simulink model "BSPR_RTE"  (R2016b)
settings: Solver=FixedStepDiscrete  StartTime=0.0  StopTime=100.0  FixedStep=0.01  RelTol=1e-3  EnableMultiTasking=on
undefined symbols (not defined in the file): RTE_bDchrgDiagStdSel_C, RTE_tiBase_C, RTE_tiDebs_C, RTE_uDCWkUpLow_C, RTE_uDCWkUpUp_C
libraries: simulink x2

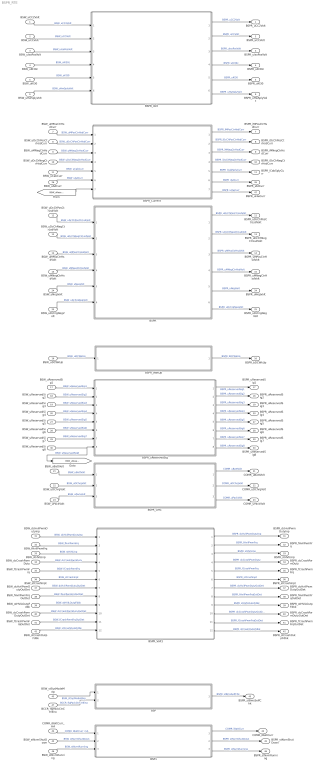
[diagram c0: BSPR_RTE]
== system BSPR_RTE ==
  BSW_uCC2Volt : Inport
  BSW_uCCVolt : Inport  Port=2
  BSW_uIsoPosVolt : Inport  Port=3
  BSW_uKl30c : Inport  Port=4
  BSW_uKl30 : Inport  Port=5
  BSW_uHwSplyVolt : Inport  Port=6
  BSW_uMPosCtrHsdCurr : Inport  Port=7
  BSW_uDcChPosCtrHsdCurr : Inport  Port=8
  BSW_uMNegCtrHsdCurr : Inport  Port=9
  BSW_uDcChNegCtrHsdCurr : Inport  Port=10
  BSW_uCabCurr : Inport  Port=11
  BSW_uDcChPosCtrLsdVolt : Inport  Port=12
  BSW_uDcChNegCtrLsdVolt : Inport  Port=13
  BSW_uMPosCtrHsdVolt : Inport  Port=14
  BSW_uMNegCtrHsdVolt : Inport  Port=15
  BSW_uDCWkUp : Inport  Port=16
  BSW_uReservedSig1 : Inport  Port=17
  BSW_uReservedSig2 : Inport  Port=18
  BSW_uReservedSig3 : Inport  Port=19
  BSW_uReservedSig4 : Inport  Port=20
  BSW_uBattVolt : Inport  Port=21
  BSW_uDChrgVolt : Inport  Port=22
  BSW_uPackVolt : Inport  Port=23
  BSW_uNegVolt : Inport  Port=24
  BSW_uDchrgNegVolt : Inport  Port=25
  BSW_uAdCurr : Inport  Port=26
  BSW_uReservedSig5 : Inport  Port=27
  BSW_uReservedSig6 : Inport  Port=28
  BSW_uReservedSig7 : Inport  Port=29
  BSW_uReservedSig8 : Inport  Port=30
  BSW_dcHvilPwmDutyInp : Inport  Port=31
  BSW_fHvilPwmFrq : Inport  Port=32
  BSW_stHVILInp : Inport  Port=33
  BSW_dcCrashPwmDuty : Inport  Port=34
  BSW_fCrashPwmFrq : Inport  Port=35
  BSW_stCrashInpt : Inport  Port=36
  BSW_dcHvilPwmDutyOutDet : Inport  Port=37
  BSW_fHvilPwmFrqOutDet : Inport  Port=38
  BSW_stHVILOutpFdbk : Inport  Port=39
  BSW_dcCrashPwmDutyOutDet : Inport  Port=40
  BSW_fCrashPwmFrqOutDet : Inport  Port=41
  BSW_stCrashOutpFdbk : Inport  Port=42
  BSW_stSysModeMag : Inport  Port=43
  " COMR_iBattCurr_mA" : Inport  Port=44
  " BSW_stNvmShutDown" : Inport  Port=45
  " BSW_stNvmRunning" : Inport  Port=46
  BCCR_flgPackCtrCtrlEna : Inport  Port=47
  BSP : Subsystem  TreatAsAtomicUnit=on
  BSP1 : Subsystem  TreatAsAtomicUnit=on
  BSPR : Subsystem  TreatAsAtomicUnit=on
  "BSPR_CMC " : Subsystem  TreatAsAtomicUnit=on
  BSPR_Current : Subsystem  TreatAsAtomicUnit=on
  BSPR_Volt : Subsystem  TreatAsAtomicUnit=on
  BSPR_Volt1 : Subsystem  TreatAsAtomicUnit=on
  BSPR_WakUp : Subsystem  TreatAsAtomicUnit=on
  BSPR_uReservedSig : Subsystem  TreatAsAtomicUnit=on
  BSPR_uCC2Volt : Outport
  BSPR_uCCVolt : Outport  Port=2
  BSPR_uIsoPosVolt : Outport  Port=3
  BSPR_uKl30c : Outport  Port=4
  BSPR_uKl30 : Outport  Port=5
  BSPR_uHwSplyVolt : Outport  Port=6
  BSPR_iMPosCtrHsdCurr : Outport  Port=7
  BSPR_iDcChPosCtrHsdCurr : Outport  Port=8
  BSPR_iMNegCtrHsdCurr : Outport  Port=9
  BSPR_iDcChNegCtrHsdCurr : Outport  Port=10
  BSPR_iCabSplyCurr : Outport  Port=11
  BSPR_uDcChPosCtrLsdVolt : Outport  Port=12
  BSPR_uDcChNegCtrLsdVolt : Outport  Port=13
  BSPR_uMPosCtrHsdVolt : Outport  Port=14
  BSPR_uMNegCtrHsdVolt : Outport  Port=15
  BSPR_bDCWkUp : Outport  Port=16
  BSPR_uReservedSig1 : Outport  Port=17
  BSPR_uReservedSig2 : Outport  Port=18
  BSPR_uReservedSig3 : Outport  Port=19
  BSPR_uReservedSig4 : Outport  Port=20
  COMR_uBattVolt : Outport  Port=21
  COMR_uDChrgVolt : Outport  Port=22
  COMR_uPackVolt : Outport  Port=23
  BSPR_uNegVolt : Outport  Port=24
  BSPR_uDchrgNegVolt : Outport  Port=25
  BSPR_iAdCurr : Outport  Port=26
  BSPR_uReservedSig5 : Outport  Port=27
  BSPR_uReservedSig6 : Outport  Port=28
  BSPR_uReservedSig7 : Outport  Port=29
  BSPR_uReservedSig8 : Outport  Port=30
  BSPR_dcHvilPwmDutyInp : Outport  Port=31
  BSPR_fHvilPwmFrq : Outport  Port=32
  BSPR_stHVILInp : Outport  Port=33
  BSPR_dcCrashPwmDuty : Outport  Port=34
  BSPR_fCrashPwmFrq : Outport  Port=35
  BSPR_stCrashInpt : Outport  Port=36
  BSPR_dcHvilPwmDutyOutDet : Outport  Port=37
  BSPR_fHvilPwmFrqOutDet : Outport  Port=38
  BSPR_stHVILOutpFdbk : Outport  Port=39
  BSPR_dcCrashPwmDutyOutDet : Outport  Port=40
  BSPR_fCrashPwmFrqOutDet : Outport  Port=41
  BSPR_stCrashOutpFdbk : Outport  Port=42
  BSPR_stBmsSelfChk : Outport  Port=43
  COMR_iBattCurr : Outport  Port=44
  BSPR_stNvmShutDown : Outport  Port=45
  BSPR_stNvmRunning : Outport  Port=46
  BSPR_uHwCurr : Outport  Port=47
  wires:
  BSW_uDcChPosCtrLsdVolt/1 -> BSPR/1(BSW_uDcChPosCtrLsdVolt)  "BSW_uDcChPosCtrLsdVolt"
  BSW_uDcChNegCtrLsdVolt/1 -> BSPR/2(BSW_uDcChNegCtrLsdVolt)  "BSW_uDcChNegCtrLsdVolt"
  BSW_uMPosCtrHsdVolt/1 -> BSPR/3(BSW_uMPosCtrHsdVolt)  "BSW_uMPosCtrHsdVolt"
  BSW_uMNegCtrHsdVolt/1 -> BSPR/4(BSW_uMNegCtrHsdVolt)  "BSW_uMNegCtrHsdVolt"
  BSPR/1(BSPR_uDcChPosCtrLsdVolt) -> BSPR_uDcChPosCtrLsdVolt/1  "BSPR_uDcChPosCtrLsdVolt"
  BSPR/2(BSPR_uDcChNegCtrLsdVolt) -> BSPR_uDcChNegCtrLsdVolt/1  "BSPR_uDcChNegCtrLsdVolt"
  BSPR/3(BSPR_uMPosCtrHsdVolt) -> BSPR_uMPosCtrHsdVolt/1  "BSPR_uMPosCtrHsdVolt"
  BSPR/4(BSPR_uMNegCtrHsdVolt) -> BSPR_uMNegCtrHsdVolt/1  "BSPR_uMNegCtrHsdVolt"
  BSW_uDCWkUp/1 -> BSPR_WakUp/1(BSW_uDCWkUp)  "BSW_uDCWkUp"
  BSPR_WakUp/1(BSPR_bDCWkUp) -> BSPR_bDCWkUp/1  "BSPR_bDCWkUp"
  BSW_uMPosCtrHsdCurr/1 -> BSPR_Current/1(BSW_uMPosCtrHsdCurr)  "BSW_uMPosCtrHsdCurr"
  BSW_uDcChPosCtrHsdCurr/1 -> BSPR_Current/2(BSW_uDcChPosCtrHsdCurr)  "BSW_uDcChPosCtrHsdCurr"
  BSW_uMNegCtrHsdCurr/1 -> BSPR_Current/3(BSW_uMNegCtrHsdCurr)  "BSW_uMNegCtrHsdCurr"
  BSW_uDcChNegCtrHsdCurr/1 -> BSPR_Current/4(BSW_uDcChNegCtrHsdCurr)  "BSW_uDcChNegCtrHsdCurr"
  BSW_uCabCurr/1 -> BSPR_Current/5(BSW_uCabCurr)  "BSW_uCabCurr"
  BSPR_Current/1(BSPR_iMPosCtrHsdCurr) -> BSPR_iMPosCtrHsdCurr/1  "BSPR_iMPosCtrHsdCurr"
  BSPR_Current/2(BSPR_iDcChPosCtrHsdCurr) -> BSPR_iDcChPosCtrHsdCurr/1  "BSPR_iDcChPosCtrHsdCurr"
  BSPR_Current/3(BSPR_iMNegCtrHsdCurr) -> BSPR_iMNegCtrHsdCurr/1  "BSPR_iMNegCtrHsdCurr"
  BSPR_Current/4(BSPR_iDcChNegCtrHsdCurr) -> BSPR_iDcChNegCtrHsdCurr/1  "BSPR_iDcChNegCtrHsdCurr"
  BSPR_Current/5(BSPR_iCabSplyCurr) -> BSPR_iCabSplyCurr/1  "BSPR_iCabSplyCurr"
  BSW_uReservedSig1/1 -> BSPR_uReservedSig/1(BSW_uReservedSig1)  "BSW_uReservedSig1"
  BSW_uReservedSig2/1 -> BSPR_uReservedSig/2(BSW_uReservedSig2)  "BSW_uReservedSig2"
  BSW_uReservedSig3/1 -> BSPR_uReservedSig/3(BSW_uReservedSig3)  "BSW_uReservedSig3"
  BSW_uReservedSig4/1 -> BSPR_uReservedSig/4(BSW_uReservedSig4)  "BSW_uReservedSig4"
  BSPR_uReservedSig/1(BSPR_uReservedSig1) -> BSPR_uReservedSig1/1  "BSPR_uReservedSig1"
  BSPR_uReservedSig/2(BSPR_uReservedSig2) -> BSPR_uReservedSig2/1  "BSPR_uReservedSig2"
  BSPR_uReservedSig/3(BSPR_uReservedSig3) -> BSPR_uReservedSig3/1  "BSPR_uReservedSig3"
  BSPR_uReservedSig/4(BSPR_uReservedSig4) -> BSPR_uReservedSig4/1  "BSPR_uReservedSig4"
  BSW_uCC2Volt/1 -> BSPR_Volt/1(BSW_uCC2Volt)  "BSW_uCC2Volt"
  BSW_uCCVolt/1 -> BSPR_Volt/2(BSW_uCCVolt)  "BSW_uCCVolt"
  BSW_uIsoPosVolt/1 -> BSPR_Volt/3(BSW_uIsoPosVolt)  "BSW_uIsoPosVolt"
  BSW_uKl30c/1 -> BSPR_Volt/4(BSW_uKl30c)  "BSW_uKl30c"
  BSW_uKl30/1 -> BSPR_Volt/5(BSW_uKl30)  "BSW_uKl30"
  BSPR_Volt/1(BSPR_uCC2Volt) -> BSPR_uCC2Volt/1  "BSPR_uCC2Volt"
  BSPR_Volt/2(BSPR_uCCVolt) -> BSPR_uCCVolt/1  "BSPR_uCCVolt"
  BSPR_Volt/3(BSPR_uIsoPosVolt) -> BSPR_uIsoPosVolt/1  "BSPR_uIsoPosVolt"
  BSPR_Volt/4(BSPR_uKl30c) -> BSPR_uKl30c/1  "BSPR_uKl30c"
  BSPR_Volt/5(BSPR_uKl30) -> BSPR_uKl30/1  "BSPR_uKl30"
  BSW_uBattVolt/1 -> "BSPR_CMC "/1(BSW_uBattVolt)  "BSW_uBattVolt"
  BSW_uDChrgVolt/1 -> "BSPR_CMC "/2(BSW_uDChrgVolt)  "BSW_uDChrgVolt"
  BSW_uPackVolt/1 -> "BSPR_CMC "/3(BSW_uPackVolt)  "BSW_uPackVolt"
  "BSPR_CMC "/1(COMR_uBattVolt) -> COMR_uBattVolt/1  "COMR_uBattVolt"
  "BSPR_CMC "/2(COMR_uDChrgVolt) -> COMR_uDChrgVolt/1  "COMR_uDChrgVolt"
  "BSPR_CMC "/3(COMR_uPackVolt) -> COMR_uPackVolt/1  "COMR_uPackVolt"
  BSW_uHwSplyVolt/1 -> BSPR_Volt/6(BSW_uHwSplyVolt)  "BSW_uHwSplyVolt"
  BSPR_Volt/6(BSPR_uHwSplyVolt) -> BSPR_uHwSplyVolt/1  "BSPR_uHwSplyVolt"
  BSW_uNegVolt/1 -> BSPR/5(BSW_uNegVolt)  "BSW_uNegVolt"
  BSW_uDchrgNegVolt/1 -> BSPR/6(BSW_uDchrgNegVolt)  "BSW_uDchrgNegVolt"
  BSPR/5(BSPR_uNegVolt) -> BSPR_uNegVolt/1  "BSPR_uNegVolt"
  BSPR/6(BSPR_uDchrgNegVolt) -> BSPR_uDchrgNegVolt/1  "BSPR_uDchrgNegVolt"
  BSPR_Current/6(BSPR_iAdCurr) -> BSPR_iAdCurr/1  "BSPR_iAdCurr"
  BSW_uAdCurr/1 -> BSPR_Current/6(BSW_uAdCurr)  "BSW_uAdCurr"
  BSW_uReservedSig5/1 -> BSPR_uReservedSig/5(BSW_uReservedSig5)  "BSW_uReservedSig5"
  BSW_uReservedSig6/1 -> BSPR_uReservedSig/6(BSW_uReservedSig6)  "BSW_uReservedSig6"
  BSW_uReservedSig7/1 -> BSPR_uReservedSig/7(BSW_uReservedSig7)  "BSW_uReservedSig7"
  BSW_uReservedSig8/1 -> [BSW_uReservedSig8], BSPR_uReservedSig/8(BSW_uReservedSig8)  "BSW_uReservedSig8"
  BSPR_uReservedSig/5(BSPR_uReservedSig5) -> BSPR_uReservedSig5/1  "BSPR_uReservedSig5"
  BSPR_uReservedSig/6(BSPR_uReservedSig6) -> BSPR_uReservedSig6/1  "BSPR_uReservedSig6"
  BSPR_uReservedSig/7(BSPR_uReservedSig7) -> BSPR_uReservedSig7/1  "BSPR_uReservedSig7"
  BSPR_uReservedSig/8(BSPR_uReservedSig8) -> BSPR_uReservedSig8/1  "BSPR_uReservedSig8"
  BSW_dcHvilPwmDutyInp/1 -> BSPR_Volt1/1(BSW_dcHvilPwmDutyInp)  "BSW_dcHvilPwmDutyInp"
  BSW_fHvilPwmFrq/1 -> BSPR_Volt1/2(BSW_fHvilPwmFrq)  "BSW_fHvilPwmFrq"
  BSW_stHVILInp/1 -> BSPR_Volt1/3(BSW_stHVILInp)  "BSW_stHVILInp"
  BSW_dcCrashPwmDuty/1 -> BSPR_Volt1/4(BSW_dcCrashPwmDuty)  "BSW_dcCrashPwmDuty"
  BSW_fCrashPwmFrq/1 -> BSPR_Volt1/5(BSW_fCrashPwmFrq)  "BSW_fCrashPwmFrq"
  BSW_stCrashInpt/1 -> BSPR_Volt1/6(BSW_stCrashInpt)  "BSW_stCrashInpt"
  BSW_dcHvilPwmDutyOutDet/1 -> BSPR_Volt1/7(BSW_dcHvilPwmDutyOutDet)  "BSW_dcHvilPwmDutyOutDet"
  BSW_fHvilPwmFrqOutDet/1 -> BSPR_Volt1/8(BSW_fHvilPwmFrqOutDet)  "BSW_fHvilPwmFrqOutDet"
  BSW_stHVILOutpFdbk/1 -> BSPR_Volt1/9(BSW_stHVILOutpFdbk)  "BSW_stHVILOutpFdbk"
  BSW_dcCrashPwmDutyOutDet/1 -> BSPR_Volt1/10(BSW_dcCrashPwmDutyOutDet)  "BSW_dcCrashPwmDutyOutDet"
  BSW_fCrashPwmFrqOutDet/1 -> BSPR_Volt1/11(BSW_fCrashPwmFrqOutDet)  "BSW_fCrashPwmFrqOutDet"
  BSW_stCrashOutpFdbk/1 -> BSPR_Volt1/12(BSW_stCrashOutpFdbk)  "BSW_stCrashOutpFdbk"
  BSPR_Volt1/1(BSPR_dcHvilPwmDutyInp) -> BSPR_dcHvilPwmDutyInp/1  "BSPR_dcHvilPwmDutyInp"
  BSPR_Volt1/2(BSPR_fHvilPwmFrq) -> BSPR_fHvilPwmFrq/1  "BSPR_fHvilPwmFrq"
  BSPR_Volt1/3(BSPR_stHVILInp) -> BSPR_stHVILInp/1  "BSPR_stHVILInp"
  BSPR_Volt1/4(BSPR_dcCrashPwmDuty) -> BSPR_dcCrashPwmDuty/1  "BSPR_dcCrashPwmDuty"
  BSPR_Volt1/5(BSPR_fCrashPwmFrq) -> BSPR_fCrashPwmFrq/1  "BSPR_fCrashPwmFrq"
  BSPR_Volt1/6(BSPR_stCrashInpt) -> BSPR_stCrashInpt/1  "BSPR_stCrashInpt"
  BSPR_Volt1/7(BSPR_dcHvilPwmDutyOutDet) -> BSPR_dcHvilPwmDutyOutDet/1  "BSPR_dcHvilPwmDutyOutDet"
  BSPR_Volt1/8(BSPR_fHvilPwmFrqOutDet) -> BSPR_fHvilPwmFrqOutDet/1  "BSPR_fHvilPwmFrqOutDet"
  BSPR_Volt1/9(BSPR_stHVILOutpFdbk) -> BSPR_stHVILOutpFdbk/1  "BSPR_stHVILOutpFdbk"
  BSPR_Volt1/10(BSPR_dcCrashPwmDutyOutDet) -> BSPR_dcCrashPwmDutyOutDet/1  "BSPR_dcCrashPwmDutyOutDet"
  BSPR_Volt1/11(BSPR_fCrashPwmFrqOutDet) -> BSPR_fCrashPwmFrqOutDet/1  "BSPR_fCrashPwmFrqOutDet"
  BSPR_Volt1/12(BSPR_stCrashOutpFdbk) -> BSPR_stCrashOutpFdbk/1  "BSPR_stCrashOutpFdbk"
  BSW_stSysModeMag/1 -> BSP/1(BSW_stSysModeMag)  "BSW_stSysModeMag"
  BSP/1(BSPR_stBmsSelfChk) -> BSPR_stBmsSelfChk/1  "BSPR_stBmsSelfChk"
  [BSW_uReservedSig8] -> BSPR_Current/7(BSW_uReservedSig8)
  " COMR_iBattCurr_mA"/1 -> BSP1/1(" COMR_iBattCurr_mA")  "COMR_iBattCurr_mA"
  BSP1/1(COMR_iBattCurr) -> COMR_iBattCurr/1  "COMR_iBattCurr"
  BSP1/2(BSPR_stNvmShutDown) -> BSPR_stNvmShutDown/1  "BSPR_stNvmShutDown"
  BSP1/3(BSPR_stNvmRunning) -> BSPR_stNvmRunning/1  "BSPR_stNvmRunning"
  " BSW_stNvmShutDown"/1 -> BSP1/2(" BSW_stNvmShutDown")  "BSW_stNvmShutDown"
  " BSW_stNvmRunning"/1 -> BSP1/3(" BSW_stNvmRunning")  "BSW_stNvmRunning"
  BCCR_flgPackCtrCtrlEna/1 -> BSP/2(BCCR_flgPackCtrCtrlEna)  "BCCR_flgPackCtrCtrlEna"
  BSPR_Current/7(BSPR_uHwCurr) -> BSPR_uHwCurr/1  "BSPR_uHwCurr"

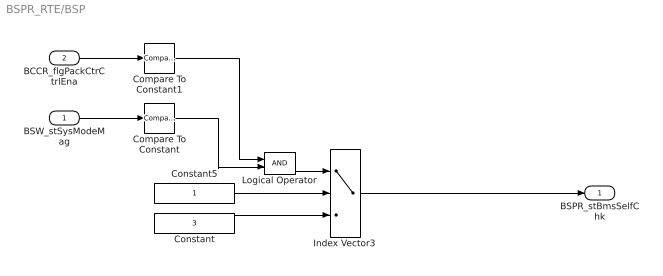
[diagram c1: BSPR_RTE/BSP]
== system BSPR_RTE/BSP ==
  BSW_stSysModeMag : Inport
  BCCR_flgPackCtrCtrlEna : Inport  Port=2
  Compare To Constant : simulink/Logic and Bit Operations/Compare To Constant  relop===  const=2  OutDataTypeStr=boolean
  Compare To Constant1 : simulink/Logic and Bit Operations/Compare To Constant  relop===  const=1  OutDataTypeStr=boolean
  Constant : Constant  Value=3  OutDataTypeStr=uint8  SampleTime=-1
  Constant5 : Constant  OutDataTypeStr=uint8  SampleTime=-1
  Index Vector3 : MultiPortSwitch  DataPortOrder=Zero-based contiguous  Inputs=2  zeroidx=on  OutDataTypeStr=uint8
  Logical Operator : Logic  AllPortsSameDT=off  OutDataTypeStr=boolean
  BSPR_stBmsSelfChk : Outport
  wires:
  Index Vector3/1 -> BSPR_stBmsSelfChk/1
  Constant/1 -> Index Vector3/3
  Constant5/1 -> Index Vector3/2
  BSW_stSysModeMag/1 -> Compare To Constant/1
  Compare To Constant/1 -> Logical Operator/2
  BCCR_flgPackCtrCtrlEna/1 -> Compare To Constant1/1
  Compare To Constant1/1 -> Logical Operator/1
  Logical Operator/1 -> Index Vector3/1

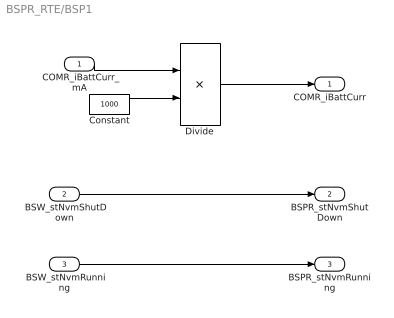
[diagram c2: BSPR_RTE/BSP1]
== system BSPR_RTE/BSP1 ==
  " COMR_iBattCurr_mA" : Inport
  " BSW_stNvmShutDown" : Inport  Port=2
  " BSW_stNvmRunning" : Inport  Port=3
  Constant : Constant  Value=1000  OutDataTypeStr=single
  Divide : Product  Inputs=*/
  COMR_iBattCurr : Outport
  BSPR_stNvmShutDown : Outport  Port=2
  BSPR_stNvmRunning : Outport  Port=3
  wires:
  " COMR_iBattCurr_mA"/1 -> Divide/1
  Constant/1 -> Divide/2
  Divide/1 -> COMR_iBattCurr/1
  " BSW_stNvmRunning"/1 -> BSPR_stNvmRunning/1
  " BSW_stNvmShutDown"/1 -> BSPR_stNvmShutDown/1

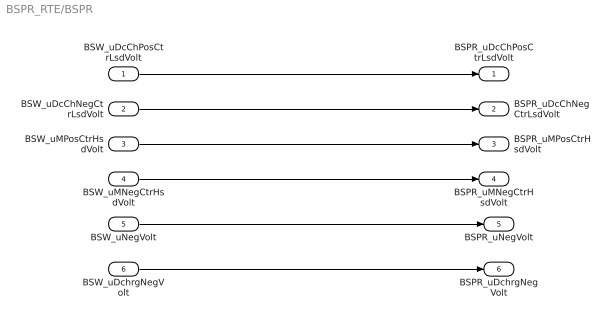
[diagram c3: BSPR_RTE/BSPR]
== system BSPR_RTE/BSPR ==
  BSW_uDcChPosCtrLsdVolt : Inport
  BSW_uDcChNegCtrLsdVolt : Inport  Port=2
  BSW_uMPosCtrHsdVolt : Inport  Port=3
  BSW_uMNegCtrHsdVolt : Inport  Port=4
  BSW_uNegVolt : Inport  Port=5
  BSW_uDchrgNegVolt : Inport  Port=6
  BSPR_uDcChPosCtrLsdVolt : Outport
  BSPR_uDcChNegCtrLsdVolt : Outport  Port=2
  BSPR_uMPosCtrHsdVolt : Outport  Port=3
  BSPR_uMNegCtrHsdVolt : Outport  Port=4
  BSPR_uNegVolt : Outport  Port=5
  BSPR_uDchrgNegVolt : Outport  Port=6
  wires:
  BSW_uDcChNegCtrLsdVolt/1 -> BSPR_uDcChNegCtrLsdVolt/1
  BSW_uMNegCtrHsdVolt/1 -> BSPR_uMNegCtrHsdVolt/1
  BSW_uDcChPosCtrLsdVolt/1 -> BSPR_uDcChPosCtrLsdVolt/1
  BSW_uMPosCtrHsdVolt/1 -> BSPR_uMPosCtrHsdVolt/1
  BSW_uNegVolt/1 -> BSPR_uNegVolt/1
  BSW_uDchrgNegVolt/1 -> BSPR_uDchrgNegVolt/1

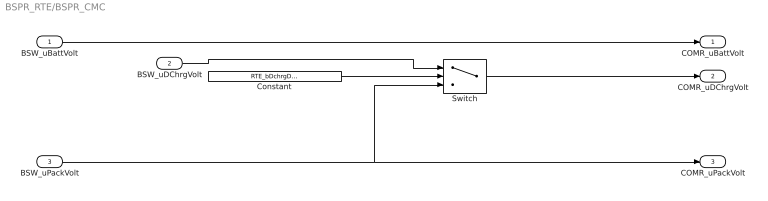
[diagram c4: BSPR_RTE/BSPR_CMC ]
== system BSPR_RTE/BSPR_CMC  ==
  BSW_uBattVolt : Inport
  BSW_uDChrgVolt : Inport  Port=2
  BSW_uPackVolt : Inport  Port=3
  Constant : Constant  Value=RTE_bDchrgDiagStdSel_C
  Switch : Switch  Criteria=u2 ~= 0
  COMR_uBattVolt : Outport  OutDataTypeStr=single
  COMR_uDChrgVolt : Outport  Port=2  OutDataTypeStr=single
  COMR_uPackVolt : Outport  Port=3  OutDataTypeStr=single
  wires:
  BSW_uBattVolt/1 -> COMR_uBattVolt/1
  BSW_uDChrgVolt/1 -> Switch/1
  BSW_uPackVolt/1 -> Switch/3, COMR_uPackVolt/1
  Constant/1 -> Switch/2
  Switch/1 -> COMR_uDChrgVolt/1

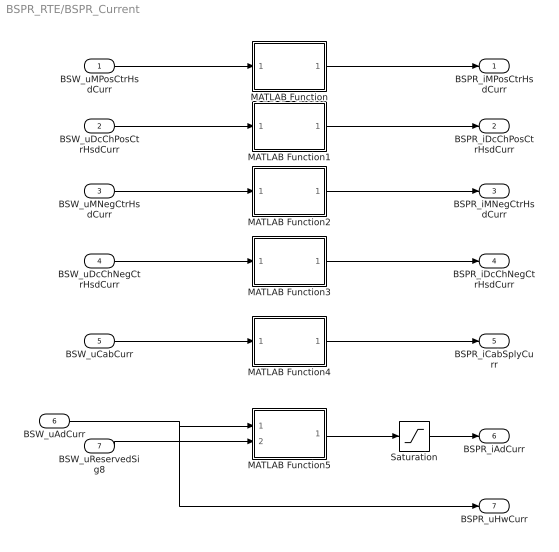
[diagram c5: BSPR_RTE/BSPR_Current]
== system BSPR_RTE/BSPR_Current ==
  BSW_uMPosCtrHsdCurr : Inport
  BSW_uDcChPosCtrHsdCurr : Inport  Port=2
  BSW_uMNegCtrHsdCurr : Inport  Port=3
  BSW_uDcChNegCtrHsdCurr : Inport  Port=4
  BSW_uCabCurr : Inport  Port=5
  BSW_uAdCurr : Inport  Port=6
  BSW_uReservedSig8 : Inport  Port=7
  MATLAB Function : MATLAB Function  TreatAsAtomicUnit=on
  MATLAB Function1 : MATLAB Function  TreatAsAtomicUnit=on
  MATLAB Function2 : MATLAB Function  TreatAsAtomicUnit=on
  MATLAB Function3 : MATLAB Function  TreatAsAtomicUnit=on
  MATLAB Function4 : MATLAB Function  TreatAsAtomicUnit=on
  MATLAB Function5 : MATLAB Function  TreatAsAtomicUnit=on
  Saturation : Saturate  UpperLimit=1024  LowerLimit=-1023
  BSPR_iMPosCtrHsdCurr : Outport
  BSPR_iDcChPosCtrHsdCurr : Outport  Port=2
  BSPR_iMNegCtrHsdCurr : Outport  Port=3
  BSPR_iDcChNegCtrHsdCurr : Outport  Port=4
  BSPR_iCabSplyCurr : Outport  Port=5
  BSPR_iAdCurr : Outport  Port=6
  BSPR_uHwCurr : Outport  Port=7
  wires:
  BSW_uMPosCtrHsdCurr/1 -> MATLAB Function/1(u)
  MATLAB Function/1(y) -> BSPR_iMPosCtrHsdCurr/1
  BSW_uDcChPosCtrHsdCurr/1 -> MATLAB Function1/1(u)
  MATLAB Function1/1(y) -> BSPR_iDcChPosCtrHsdCurr/1
  BSW_uMNegCtrHsdCurr/1 -> MATLAB Function2/1(u)
  MATLAB Function2/1(y) -> BSPR_iMNegCtrHsdCurr/1
  BSW_uDcChNegCtrHsdCurr/1 -> MATLAB Function3/1(u)
  MATLAB Function3/1(y) -> BSPR_iDcChNegCtrHsdCurr/1
  BSW_uCabCurr/1 -> MATLAB Function4/1(u)
  MATLAB Function4/1(y) -> BSPR_iCabSplyCurr/1
  BSW_uAdCurr/1 -> BSPR_uHwCurr/1, MATLAB Function5/1(u)
  MATLAB Function5/1(y) -> Saturation/1
  BSW_uReservedSig8/1 -> MATLAB Function5/2(v)
  Saturation/1 -> BSPR_iAdCurr/1

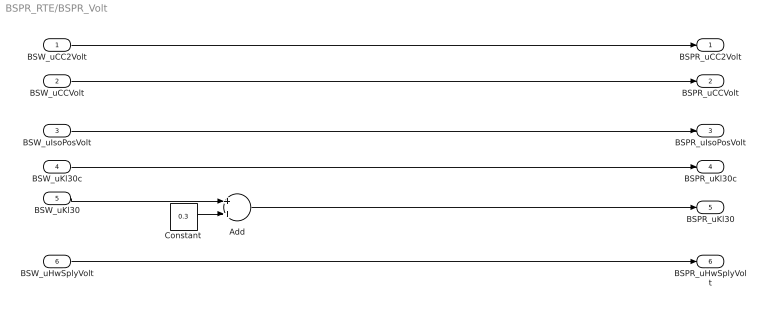
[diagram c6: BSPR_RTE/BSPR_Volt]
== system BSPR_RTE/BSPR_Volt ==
  BSW_uCC2Volt : Inport
  BSW_uCCVolt : Inport  Port=2
  BSW_uIsoPosVolt : Inport  Port=3
  BSW_uKl30c : Inport  Port=4
  BSW_uKl30 : Inport  Port=5
  BSW_uHwSplyVolt : Inport  Port=6
  Add : Sum  OutDataTypeStr=single
  Constant : Constant  Value=0.3  OutDataTypeStr=single
  BSPR_uCC2Volt : Outport
  BSPR_uCCVolt : Outport  Port=2
  BSPR_uIsoPosVolt : Outport  Port=3
  BSPR_uKl30c : Outport  Port=4
  BSPR_uKl30 : Outport  Port=5
  BSPR_uHwSplyVolt : Outport  Port=6
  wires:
  BSW_uCC2Volt/1 -> BSPR_uCC2Volt/1
  BSW_uIsoPosVolt/1 -> BSPR_uIsoPosVolt/1
  BSW_uKl30c/1 -> BSPR_uKl30c/1
  BSW_uKl30/1 -> Add/1
  BSW_uCCVolt/1 -> BSPR_uCCVolt/1
  BSW_uHwSplyVolt/1 -> BSPR_uHwSplyVolt/1
  Constant/1 -> Add/2
  Add/1 -> BSPR_uKl30/1

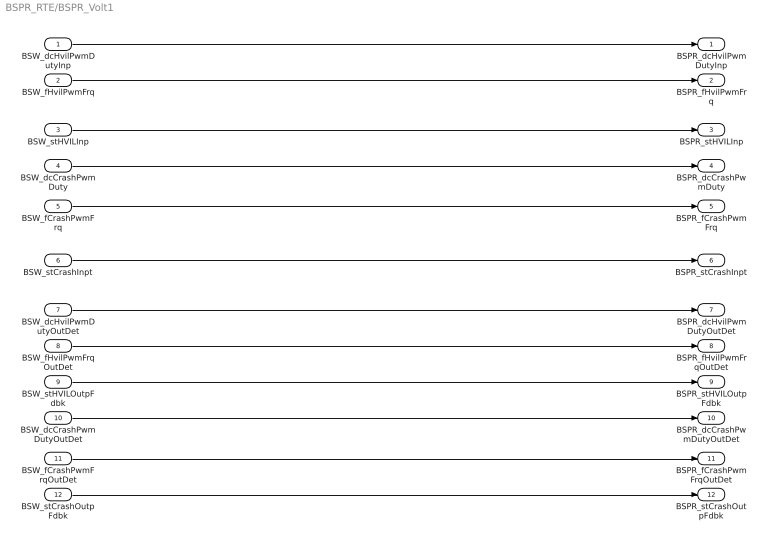
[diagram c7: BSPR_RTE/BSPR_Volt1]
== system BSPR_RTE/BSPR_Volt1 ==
  BSW_dcHvilPwmDutyInp : Inport
  BSW_fHvilPwmFrq : Inport  Port=2
  BSW_stHVILInp : Inport  Port=3
  BSW_dcCrashPwmDuty : Inport  Port=4
  BSW_fCrashPwmFrq : Inport  Port=5
  BSW_stCrashInpt : Inport  Port=6
  BSW_dcHvilPwmDutyOutDet : Inport  Port=7
  BSW_fHvilPwmFrqOutDet : Inport  Port=8
  BSW_stHVILOutpFdbk : Inport  Port=9
  BSW_dcCrashPwmDutyOutDet : Inport  Port=10
  BSW_fCrashPwmFrqOutDet : Inport  Port=11
  BSW_stCrashOutpFdbk : Inport  Port=12
  BSPR_dcHvilPwmDutyInp : Outport
  BSPR_fHvilPwmFrq : Outport  Port=2
  BSPR_stHVILInp : Outport  Port=3
  BSPR_dcCrashPwmDuty : Outport  Port=4
  BSPR_fCrashPwmFrq : Outport  Port=5
  BSPR_stCrashInpt : Outport  Port=6
  BSPR_dcHvilPwmDutyOutDet : Outport  Port=7
  BSPR_fHvilPwmFrqOutDet : Outport  Port=8
  BSPR_stHVILOutpFdbk : Outport  Port=9
  BSPR_dcCrashPwmDutyOutDet : Outport  Port=10
  BSPR_fCrashPwmFrqOutDet : Outport  Port=11
  BSPR_stCrashOutpFdbk : Outport  Port=12
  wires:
  BSW_dcCrashPwmDutyOutDet/1 -> BSPR_dcCrashPwmDutyOutDet/1
  BSW_stHVILOutpFdbk/1 -> BSPR_stHVILOutpFdbk/1
  BSW_fHvilPwmFrqOutDet/1 -> BSPR_fHvilPwmFrqOutDet/1
  BSW_dcHvilPwmDutyOutDet/1 -> BSPR_dcHvilPwmDutyOutDet/1
  BSW_fHvilPwmFrq/1 -> BSPR_fHvilPwmFrq/1
  BSW_fCrashPwmFrq/1 -> BSPR_fCrashPwmFrq/1
  BSW_dcCrashPwmDuty/1 -> BSPR_dcCrashPwmDuty/1
  BSW_stHVILInp/1 -> BSPR_stHVILInp/1
  BSW_dcHvilPwmDutyInp/1 -> BSPR_dcHvilPwmDutyInp/1
  BSW_fCrashPwmFrqOutDet/1 -> BSPR_fCrashPwmFrqOutDet/1
  BSW_stCrashOutpFdbk/1 -> BSPR_stCrashOutpFdbk/1
  BSW_stCrashInpt/1 -> BSPR_stCrashInpt/1

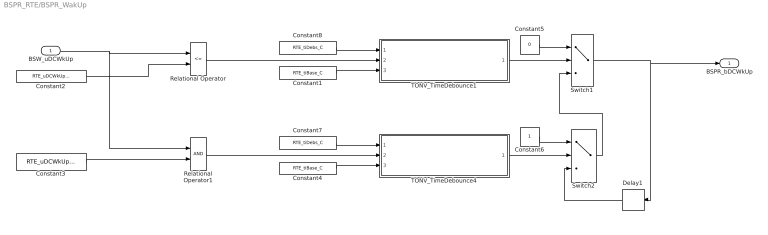
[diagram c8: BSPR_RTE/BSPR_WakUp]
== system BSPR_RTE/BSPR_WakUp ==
  BSW_uDCWkUp : Inport
  Constant1 : Constant  Value=RTE_tiBase_C
  Constant2 : Constant  Value=RTE_uDCWkUpLow_C  OutDataTypeStr=single
  Constant3 : Constant  Value=RTE_uDCWkUpUp_C  OutDataTypeStr=single
  Constant4 : Constant  Value=RTE_tiBase_C
  Constant5 : Constant  Value=0  OutDataTypeStr=boolean
  Constant6 : Constant  OutDataTypeStr=boolean
  Constant7 : Constant  Value=RTE_tiDebs_C
  Constant8 : Constant  Value=RTE_tiDebs_C
  Delay1 : Delay  DelayLength=1  InitialCondition=0
  Relational Operator : RelationalOperator  Operator=<=  OutDataTypeStr=boolean  RndMeth=Simplest
  Relational Operator1 : RelationalOperator  OutDataTypeStr=boolean  RndMeth=Simplest
  Switch1 : Switch  Criteria=u2 > Threshold
  Switch2 : Switch  Criteria=u2 > Threshold
  TONV_TimeDebounce1 : Subsystem  TreatAsAtomicUnit=on
  TONV_TimeDebounce4 : Subsystem  TreatAsAtomicUnit=on
  BSPR_bDCWkUp : Outport
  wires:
  Constant6/1 -> Switch2/1
  BSW_uDCWkUp/1 -> Relational Operator1/1, Relational Operator/1
  Constant2/1 -> Relational Operator/2
  Constant5/1 -> Switch1/1
  Constant3/1 -> Relational Operator1/2
  Switch2/1 -> Switch1/3
  Delay1/1 -> Switch2/3
  Switch1/1 -> BSPR_bDCWkUp/1, Delay1/1
  TONV_TimeDebounce4/1(y) -> Switch2/2
  Constant4/1 -> TONV_TimeDebounce4/3(dT)
  Constant7/1 -> TONV_TimeDebounce4/1(T)
  Relational Operator1/1 -> TONV_TimeDebounce4/2(u)
  TONV_TimeDebounce1/1(y) -> Switch1/2
  Constant1/1 -> TONV_TimeDebounce1/3(dT)
  Constant8/1 -> TONV_TimeDebounce1/1(T)
  Relational Operator/1 -> TONV_TimeDebounce1/2(u)

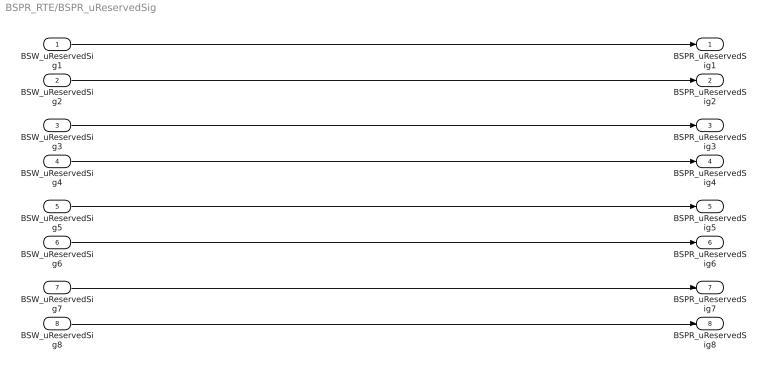
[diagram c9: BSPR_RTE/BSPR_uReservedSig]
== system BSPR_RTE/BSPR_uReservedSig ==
  BSW_uReservedSig1 : Inport
  BSW_uReservedSig2 : Inport  Port=2
  BSW_uReservedSig3 : Inport  Port=3
  BSW_uReservedSig4 : Inport  Port=4
  BSW_uReservedSig5 : Inport  Port=5
  BSW_uReservedSig6 : Inport  Port=6
  BSW_uReservedSig7 : Inport  Port=7
  BSW_uReservedSig8 : Inport  Port=8
  BSPR_uReservedSig1 : Outport
  BSPR_uReservedSig2 : Outport  Port=2
  BSPR_uReservedSig3 : Outport  Port=3
  BSPR_uReservedSig4 : Outport  Port=4
  BSPR_uReservedSig5 : Outport  Port=5
  BSPR_uReservedSig6 : Outport  Port=6
  BSPR_uReservedSig7 : Outport  Port=7
  BSPR_uReservedSig8 : Outport  Port=8
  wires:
  BSW_uReservedSig1/1 -> BSPR_uReservedSig1/1
  BSW_uReservedSig2/1 -> BSPR_uReservedSig2/1
  BSW_uReservedSig3/1 -> BSPR_uReservedSig3/1
  BSW_uReservedSig4/1 -> BSPR_uReservedSig4/1
  BSW_uReservedSig5/1 -> BSPR_uReservedSig5/1
  BSW_uReservedSig6/1 -> BSPR_uReservedSig6/1
  BSW_uReservedSig7/1 -> BSPR_uReservedSig7/1
  BSW_uReservedSig8/1 -> BSPR_uReservedSig8/1

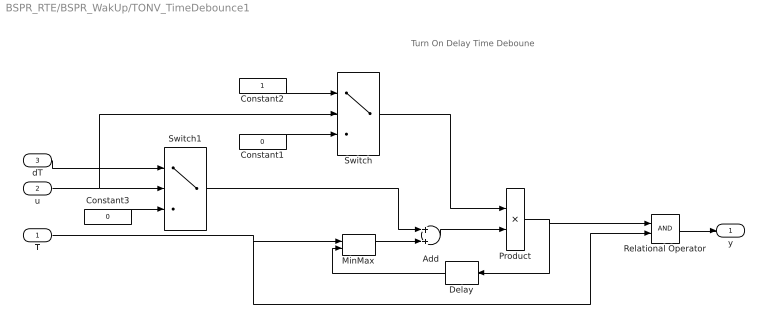
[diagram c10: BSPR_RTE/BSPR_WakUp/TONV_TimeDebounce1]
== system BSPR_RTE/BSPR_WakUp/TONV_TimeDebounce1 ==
  note: Turn On Delay Time Deboune
  T : Inport
  u : Inport  Port=2
  dT : Inport  Port=3
  Add : Sum
  Constant1 : Constant  Value=0  OutDataTypeStr=uint8
  Constant2 : Constant  OutDataTypeStr=uint8
  Constant3 : Constant  Value=0  OutDataTypeStr=single
  Delay : Delay  DelayLength=1  InitialCondition=0
  MinMax : MinMax  Inputs=2
  Product : Product  OutMin=[0]  OutMax=[65535]  OutDataTypeStr=single
  Relational Operator : RelationalOperator  OutDataTypeStr=boolean  RndMeth=Simplest
  Switch : Switch  Criteria=u2 ~= 0
  Switch1 : Switch  Criteria=u2 ~= 0
  y : Outport
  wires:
  MinMax/1 -> Add/2
  T/1 -> MinMax/1, Relational Operator/2
  Relational Operator/1 -> y/1
  Delay/1 -> MinMax/2
  Switch1/1 -> Add/1
  Product/1 -> Delay/1, Relational Operator/1
  Add/1 -> Product/2
  Constant1/1 -> Switch/3
  Constant2/1 -> Switch/1
  Constant3/1 -> Switch1/3
  dT/1 -> Switch1/1
  Switch/1 -> Product/1
  u/1 -> Switch/2, Switch1/2

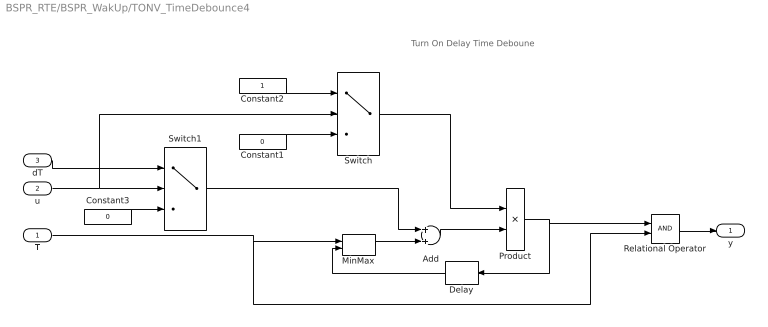
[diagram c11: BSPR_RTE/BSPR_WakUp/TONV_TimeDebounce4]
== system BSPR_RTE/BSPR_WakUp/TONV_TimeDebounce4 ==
  note: Turn On Delay Time Deboune
  T : Inport
  u : Inport  Port=2
  dT : Inport  Port=3
  Add : Sum
  Constant1 : Constant  Value=0  OutDataTypeStr=uint8
  Constant2 : Constant  OutDataTypeStr=uint8
  Constant3 : Constant  Value=0  OutDataTypeStr=single
  Delay : Delay  DelayLength=1  InitialCondition=0
  MinMax : MinMax  Inputs=2
  Product : Product  OutMin=[0]  OutMax=[65535]  OutDataTypeStr=single
  Relational Operator : RelationalOperator  OutDataTypeStr=boolean  RndMeth=Simplest
  Switch : Switch  Criteria=u2 ~= 0
  Switch1 : Switch  Criteria=u2 ~= 0
  y : Outport
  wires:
  u/1 -> Switch1/2, Switch/2
  Switch/1 -> Product/1
  dT/1 -> Switch1/1
  Constant3/1 -> Switch1/3
  Constant2/1 -> Switch/1
  Constant1/1 -> Switch/3
  Add/1 -> Product/2
  Product/1 -> Relational Operator/1, Delay/1
  Switch1/1 -> Add/1
  Delay/1 -> MinMax/2
  Relational Operator/1 -> y/1
  T/1 -> Relational Operator/2, MinMax/1
  MinMax/1 -> Add/2

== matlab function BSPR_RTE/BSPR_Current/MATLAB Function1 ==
function y=fcn(u)
u=u/1000;
if (u<0.04)
  y=0.05/0.04*u;
elseif (u<=1.16)
  y=0.05+(1-0.05)/(1.16-0.04)*(u-0.04);
elseif (u<=2.44)
  y=1+(2-1)/(2.44-1.16)*(u-1.16);
elseif (u<=4.94)
  y=2+(4-2)/(4.94-2.44)*(u-2.44);
else 
  y=u/2150*1740;
end

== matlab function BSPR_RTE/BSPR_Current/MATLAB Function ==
function y=fcn(u)
u=u/1000;
if (u<0.04)
  y=0.05/0.04*u;
elseif (u<=1.16)
  y=0.05+(1-0.05)/(1.16-0.04)*(u-0.04);
elseif (u<=2.44)
  y=1+(2-1)/(2.44-1.16)*(u-1.16);
elseif (u<=4.94)
  y=2+(4-2)/(4.94-2.44)*(u-2.44);
else 
  y=u/2150*1740;
end

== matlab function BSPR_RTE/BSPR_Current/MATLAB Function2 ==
function y=fcn(u)
u=u/1000;
if (u<0.04)
  y=0.05/0.04*u;
elseif (u<=1.16)
  y=0.05+(1-0.05)/(1.16-0.04)*(u-0.04);
elseif (u<=2.44)
  y=1+(2-1)/(2.44-1.16)*(u-1.16);
elseif (u<=4.94)
  y=2+(4-2)/(4.94-2.44)*(u-2.44);
else 
  y=u/2150*1740;
end

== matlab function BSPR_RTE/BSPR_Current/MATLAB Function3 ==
function y=fcn(u)
u=u/1000;
if (u<0.04)
  y=0.05/0.04*u;
elseif (u<=1.16)
  y=0.05+(1-0.05)/(1.16-0.04)*(u-0.04);
elseif (u<=2.44)
  y=1+(2-1)/(2.44-1.16)*(u-1.16);
elseif (u<=4.94)
  y=2+(4-2)/(4.94-2.44)*(u-2.44);
else 
  y=u/2150*1740;
end

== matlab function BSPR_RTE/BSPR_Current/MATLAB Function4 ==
function y=fcn(u)
u=u/1000;
if (u<0.05)
  y=0.001*u*500;
elseif (u<=0.78)
  y=0.001*u*450;
else 
  y=0.001*u*440;
end

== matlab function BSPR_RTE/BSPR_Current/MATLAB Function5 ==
function y=fcn(u,v)
y=(u/(v/5)-2.5)/0.002;
